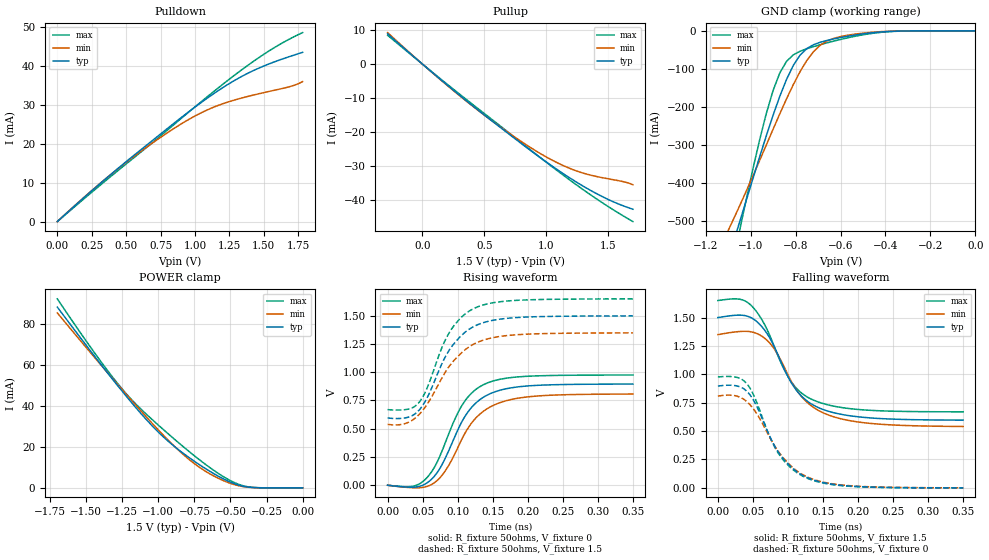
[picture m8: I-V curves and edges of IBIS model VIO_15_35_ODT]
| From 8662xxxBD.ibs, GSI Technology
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[Model]   VIO_15_35_ODT
Model_type   I/O
Polarity   Non-Inverting
Vinl  =   0.5500V
Vinh  =   0.9500V
Vmeas =   0.75v
Rref  =   50
|  variable   typ   min   max
C_comp   3.0pF   2.5pF   3.5pF
[Receiver Thresholds]
Vth = 0.75V
Vth_min = 0.68V
Vth_max = 0.825V
Threshold_sensitivity = 1.0
Reference_supply Ext_ref
Vinh_ac = +200mv
Vinh_dc = +100mv
Vinl_ac = -200mv
Vinl_dc = -100mv
Tslew_ac = 550ps
|  variable   typ   min   max
[External Reference]   0.75   0.68   0.825
|  variable   typ   min   max
[Temperature Range]   50   100   0
|  variable   typ   min   max
[Voltage Range]   1.5   1.35   1.65
[Add Submodel]
| Submodel Name   Mode
Strong_ODT_15V   Non-Driving
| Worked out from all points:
|   slope of the pulldown table from 0 to 0.225 V, typ, clamps not added: 31.6 ohm
|   slope of the pullup table from 0 to 0.225 V, typ, clamps not added: 32.5 ohm
|   GND clamp passes 1 mA (typ) near -0.36 V on its own axis
|   POWER clamp passes 1 mA (typ) near -0.42 V on its own axis
|   rising waveform, R_fixture 50ohms, V_fixture 0: 20-80 % time 46.7ps typ, 49.1ps min, 44.8ps max; typ from 0 V to 0.896 V
|   rising waveform, R_fixture 50ohms, V_fixture 1.5: 20-80 % time 47.7ps typ, 53.6ps min, 43.6ps max; typ from 0.595 V to 1.5 V
|   falling waveform, R_fixture 50ohms, V_fixture 1.5: 20-80 % time 50.7ps typ, 54ps min, 48.6ps max; typ from 1.5 V to 0.596 V
|   falling waveform, R_fixture 50ohms, V_fixture 0: 20-80 % time 49.7ps typ, 54ps min, 47.4ps max; typ from 0.897 V to 0 V
[Pullup]
| V(VDDQ-Vout)   typ   min   max
-280mV    8.881mA    9.249mA    8.449mA
60mV      -1.871mA   -1.919mA   -1.794mA
360mV     -10.95mA   -11.08mA   -10.59mA
640mV     -18.97mA   -18.81mA   -18.56mA
900mV     -26.19mA   -25.22mA   -26.08mA
1.08V     -30.89mA   -28.92mA   -31.16mA
1.24V     -34.7mA    -31.45mA   -35.49mA
1.34V     -36.86mA   -32.57mA   -38.08mA
1.48V     -39.55mA   -33.68mA   -41.52mA
1.62V     -41.76mA   -34.65mA   -44.71mA
1.7V      -42.78mA   -35.58mA   -46.42mA
[PullDown]
| voltage   typ   min   max
0V        -6.62nA    -14.14nA   -2.867nA
252mV     7.949mA    8.017mA    7.573mA
486mV     14.96mA    14.82mA    14.38mA
738mV     22.13mA    21.31mA    21.63mA
954mV     28.14mA    26.18mA    28.06mA
1.134V    32.76mA    29.32mA    33.3mA
1.242V    35.24mA    30.69mA    36.32mA
1.35V     37.43mA    31.79mA    39.2mA
1.458V    39.27mA    32.74mA    41.91mA
1.566V    40.83mA    33.6mA     44.39mA
1.71V     42.6mA     34.84mA    47.25mA
1.782V    43.42mA    35.92mA    48.48mA
[POWER Clamp]
|V(VDDQ-Vout)   typ   min   max
-1.7V     88.47mA    85.63mA    92.51mA
-1.428V   63.15mA    62.67mA    64.71mA
-1.224V   45.01mA    45.89mA    46.19mA
-1.122V   36.5mA     37.74mA    38.64mA
-1.02V    28.71mA    29.85mA    31.98mA
-918mV    21.99mA    22.38mA    25.61mA
-816mV    16.3mA     15.63mA    19.48mA
-646mV    8.221mA    6.972mA    10.07mA
-544mV    4.192mA    3.378mA    5.259mA
-442mV    1.292mA    1.001mA    1.675mA
-340mV    147uA      124.8uA    177uA
0V        29.63nA    52.34nA    12.42nA
[GND Clamp]
|(Vout)   typ   min   max
-1.5V     -1.252A    -991.4mA   -1.695A
-1.11V    -618mA     -537.1mA   -698.9mA
-1.08V    -561.6mA   -499.5mA   -613mA
-1.05V    -504.3mA   -461mA     -527.9mA
-930mV    -275.4mA   -299.5mA   -216.7mA
-900mV    -221.7mA   -258.3mA   -156.7mA
-870mV    -171.8mA   -217.7mA   -110.4mA
-810mV    -90.75mA   -141.1mA   -63.05mA
-720mV    -36.4mA    -54.51mA   -41.47mA
-630mV    -21.2mA    -19.75mA   -26.98mA
-390mV    -1.825mA   -1.274mA   -2.426mA
0V        -6.62nA    -14.14nA   -2.873nA
[Ramp]
| voltage   typ   min   max
dV/dt_r   0.54/186p   0.48/213p   0.60/209p
dV/dt_f   0.86/129p   0.66/166p   1.07/101p
R_load  =   50ohms
[Rising Waveform]
R_fixture =   50ohms
V_fixture =   0
| Time   V(typ)   V(min)   V(max)
0s        126.8nV    266.9nV    56.82nV
38.5ps    -16.56mV   -22.71mV   -5.499mV
63ps      54.93mV    7.782mV    121.3mV
84ps      262.1mV    143.6mV    403.8mV
105ps     551.7mV    397.1mV    695.4mV
119ps     683.4mV    544mV      810.5mV
140ps     790.7mV    669.1mV    899mV
168ps     852.4mV    746mV      946.1mV
203ps     880.1mV    783.9mV    965.4mV
350ps     895.5mV    807.1mV    975.7mV
[Rising Waveform]
R_fixture =   50ohms
V_fixture =   1.5
V_fixture_min =  1.35
V_fixture_max =  1.65
| Time   V(typ)   V(min)   V(max)
0s        595.4mV    538.3mV    669.3mV
24.5ps    595.4mV    544.8mV    668.7mV
45.5ps    668.3mV    629.6mV    737.6mV
56ps      769.3mV    712.9mV    855.5mV
77ps      1.069V     943.8mV    1.21V
87.5ps    1.192V     1.049V     1.346V
105ps     1.323V     1.169V     1.485V
126ps     1.414V     1.258V     1.572V
185.5ps   1.484V     1.332V     1.637V
350ps     1.499V     1.348V     1.649V
[Falling Waveform]
R_fixture =   50ohms
V_fixture =   1.5
V_fixture_min = 1.35
V_fixture_max = 1.65
| Time   V(typ)   V(min)   V(max)
0s        1.5V       1.35V      1.65V
38.5ps    1.517V     1.379V     1.647V
66.5ps    1.391V     1.319V     1.441V
80.5ps    1.243V     1.224V     1.244V
101.5ps   961.8mV    976.6mV    964.7mV
115.5ps   833.6mV    833.9mV    856mV
133ps     740.6mV    724.3mV    782.2mV
161ps     668.9mV    634.4mV    725.4mV
199.5ps   626.3mV    580.8mV    690.9mV
350ps     596.4mV    540.5mV    669.6mV
[Falling Waveform]
R_fixture =   50ohms
V_fixture =   0
| Time   V(typ)   V(min)   V(max)
0s        896.8mV    808.8mV    976.5mV
28ps      896.4mV    806.4mV    971.6mV
42ps      846.8mV    756.1mV    912mV
52.5ps    754.5mV    680.5mV    797.9mV
73.5ps    459.9mV    450.7mV    456.9mV
84ps      337mV      340.8mV    327.2mV
105ps     180.8mV    189mV      171.4mV
126ps     94.63mV    100.5mV    88.57mV
189ps     15.98mV    18.7mV     13.39mV
350ps     242.8uV    468.6uV    116.8uV
